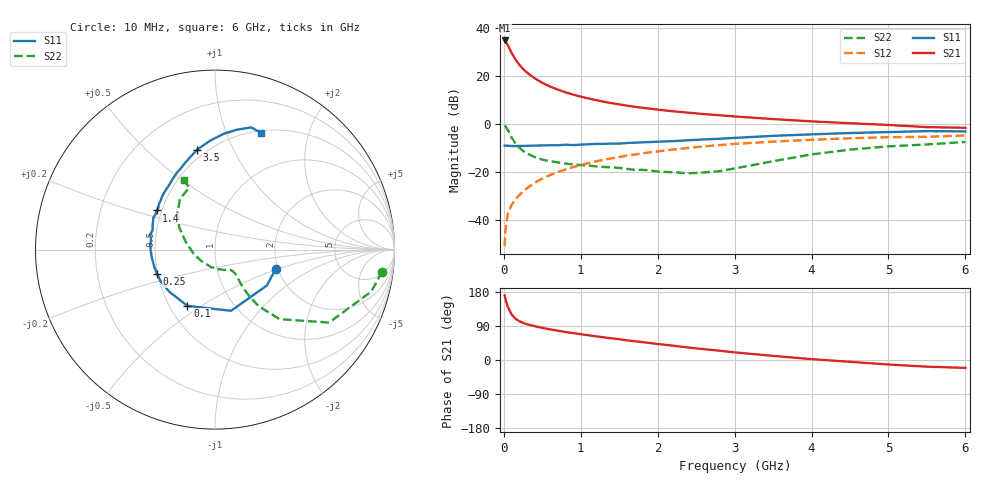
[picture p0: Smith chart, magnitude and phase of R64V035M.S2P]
! SIEMENS Small Signal Semiconductors
! BFR193
! Si NPN RF Bipolar Junction Transistor in SOT23
! VCE = 4 V  IC = 35 mA
! Common Emitter S-Parameters:  May  1996
# GHz  S  MA  R  50
!  f  S11  S21  S12  S22
! GHz  MAG  ANG  MAG  ANG  MAG  ANG  MAG  ANG
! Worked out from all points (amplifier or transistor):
!   36 points, 10 MHz to 6 GHz, reference 50 ohm
!   highest |S21| = 34.7 dB at 10 MHz (marker M1)
!   |S21| within 3 dB of that: start of sweep to 67.74 MHz
!   unconditionally stable (mu >= 1): 458.1 MHz to 1.914 GHz
!   at 250 MHz: K = 0.92, MSG = 25.4 dB, |S12| = -28.0 dB
!   at 1.4 GHz: K = 1.02, MAG = 10.6 dB, |S12| = -14.3 dB
!   at 6 GHz: K = 0.95, MSG = 1.6 dB, |S12| = -4.8 dB
!   S11 on the Smith chart (normalised r, x): 10 MHz: 1.95, -0.48; 100 MHz: 0.61, -0.44; 250 MHz: 0.50, -0.15; 1.4 GHz: 0.47, +0.24; 3.5 GHz: 0.45, +0.73; 6 GHz: 0.52, +1.34
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0.01  0.3554 -17.5  54.18 170.7  0.0029 80.7  0.9386 -7.5
0.02  0.3514 -34.7  52.45 161.9  0.0059 82.1  0.9018 -15.0
0.05  0.3525 -75.3  43.86 140.9  0.0133 71.1  0.7547 -32.6
0.1  0.3492 -116.2  30.06 120.5  0.0207 68.0  0.5281 -47.2
0.15  0.3463 -137.4  21.93 109.1  0.0272 67.2  0.3986 -52.3
0.2  0.3506 -149.6  17.08 102.5  0.0332 69.7  0.323 -53.6
0.25  0.3497 -157.2  13.87 97.8  0.0398 70.7  0.275 -53.7
0.3  0.3513 -163.6  11.68 94.4  0.0463 71.3  0.2446 -53.1
0.4  0.3552 -172.9  8.907 89.3  0.0598 72.8  0.2055 -51.6
0.5  0.3579 -179.0  7.149 84.7  0.0732 72.8  0.1816 -50.3
0.6  0.3614 175.9  6.004 80.9  0.0868 72.5  0.1692 -50.0
0.7  0.3608 171.0  5.185 77.3  0.1 71.7  0.1594 -50.5
0.8  0.371 166.8  4.55 74.0  0.1133 70.7  0.1506 -51.3
0.9  0.364 162.8  4.068 71.0  0.1275 69.7  0.1442 -52.0
1.1  0.378 156.0  3.385 65.2  0.1538 67.4  0.1362 -56.4
1.4  0.3912 146.1  2.701 57.2  0.1935 63.6  0.1261 -64.2
1.7  0.4074 138.0  2.277 49.5  0.2319 59.4  0.1118 -75.6
2.2  0.4397 125.8  1.833 37.7  0.2946 52.1  0.0994 -103.9
3.5  0.5662 100.1  1.263 10.9  0.4294 31.9  0.1684 165.3
4.5  0.6482 85.5  1.036 -4.8  0.5043 17.8  0.2927 135.5
5.5  0.7099 73.6  0.859 -17.6  0.5413 3.9  0.3753 112.4
6  0.7002 68.3  0.834 -20.8  0.5771 -0.1  0.4231 114.5
